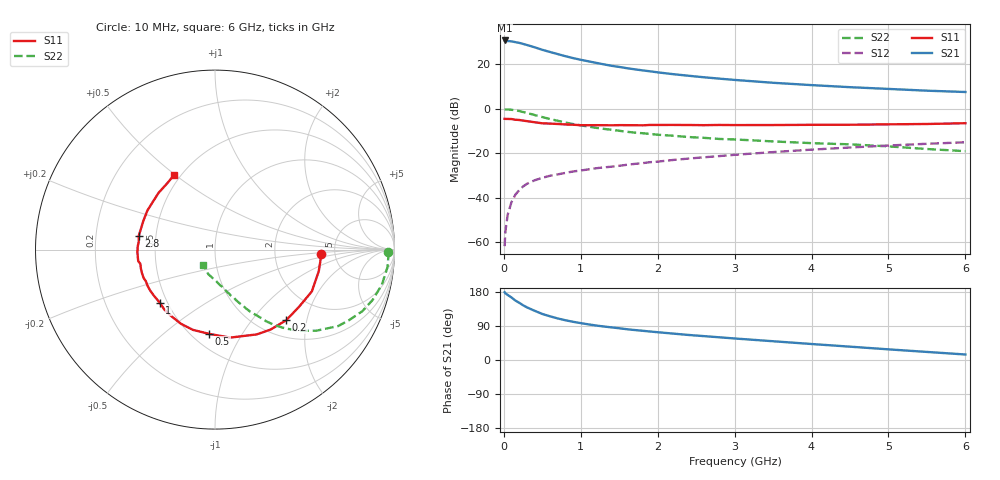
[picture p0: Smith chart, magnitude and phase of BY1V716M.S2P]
! SIEMENS Small Signal Semiconductors
! BFY420
! Si NPN RF SIEGET Grounded Emitter Transistor in MICRO-X
! VCE = 1.75 V  IC = 16 mA
! Common Emitter S-Parameters:  October  1996
# GHz  S  MA  R  50
!  f  S11  S21  S12  S22
! GHz  MAG  ANG  MAG  ANG  MAG  ANG  MAG  ANG
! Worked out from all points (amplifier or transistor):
!   36 points, 10 MHz to 6 GHz, reference 50 ohm
!   highest |S21| = 30.8 dB at 10 MHz (marker M1)
!   |S21| within 3 dB of that: start of sweep to 392.5 MHz
!   unconditionally stable (mu >= 1): 2.093 GHz to end of sweep
!   at 250 MHz: K = 0.26, MSG = 32.1 dB, |S12| = -35.0 dB
!   at 1.4 GHz: K = 0.88, MSG = 22.7 dB, |S12| = -26.1 dB
!   at 6 GHz: K = 1.09, MAG = 9.5 dB, |S12| = -15.1 dB
!   S11 on the Smith chart (normalised r, x): 10 MHz: 3.90, -0.32; 200 MHz: 1.32, -1.52; 500 MHz: 0.60, -0.73; 1 GHz: 0.45, -0.33; 2.8 GHz: 0.40, +0.07; 6 GHz: 0.46, +0.49
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0.01  0.5939 -2.6  34.7 178.8  0.0008 104.4  0.9644 -0.7
0.02  0.5913 -4.9  34.6 176.0  0.0017 87.2  0.967 -1.9
0.05  0.5906 -11.8  33.64 171.7  0.0041 86.7  0.9662 -5.8
0.1  0.5877 -23.4  33.1 164.9  0.0079 81.5  0.95 -11.9
0.15  0.5665 -34.2  31.78 156.9  0.0116 75.0  0.9221 -17.7
0.2  0.5588 -44.8  30.62 151.0  0.0147 73.0  0.8896 -22.7
0.25  0.5426 -55.2  29 144.4  0.0177 67.5  0.8454 -27.6
0.3  0.5266 -63.8  27.41 138.9  0.0204 65.3  0.808 -31.8
0.4  0.4976 -80.2  24.34 129.9  0.0244 61.4  0.7229 -38.7
0.5  0.4707 -94.0  21.35 121.5  0.0278 57.9  0.6502 -44.1
0.6  0.4638 -105.5  19.1 115.3  0.0309 56.2  0.5877 -48.3
0.7  0.4549 -114.6  17.11 109.7  0.0332 55.4  0.5367 -51.7
0.8  0.4433 -123.6  15.35 104.9  0.0359 53.7  0.4901 -54.5
1  0.4268 -136.2  12.73 97.3  0.0407 53.5  0.4233 -58.4
1.1  0.4264 -142.5  11.74 94.0  0.043 53.7  0.3965 -60.5
1.6  0.4273 -162.4  8.217 81.2  0.0547 53.3  0.3035 -67.5
2.2  0.4325 -177.9  6.029 69.7  0.0702 52.4  0.2468 -73.9
2.8  0.4321 170.0  4.786 59.9  0.0858 49.8  0.2089 -79.6
3.5  0.4302 157.9  3.856 49.5  0.1056 45.5  0.1839 -85.8
4.5  0.437 142.1  3.069 35.2  0.134 37.9  0.1579 -95.5
5.5  0.4544 126.3  2.559 21.3  0.1626 28.8  0.1239 -113.8
6  0.4726 119.1  2.389 14.5  0.1759 24.1  0.1108 -127.4
